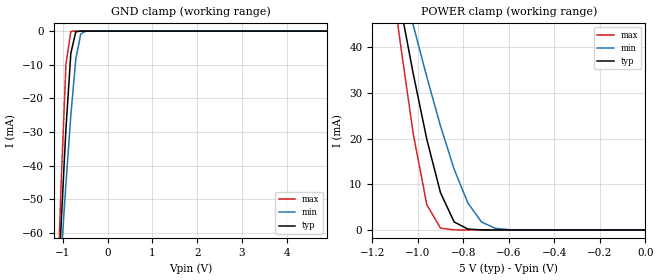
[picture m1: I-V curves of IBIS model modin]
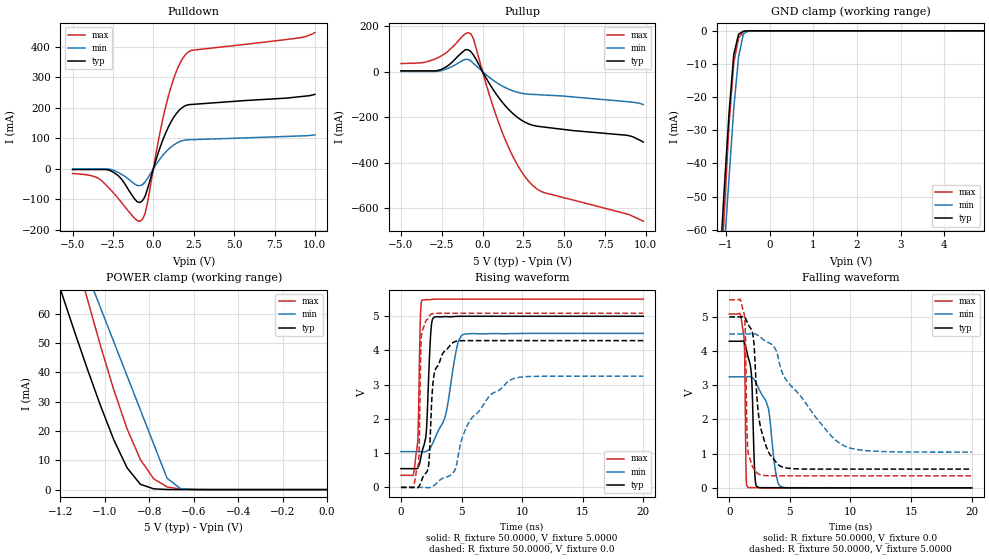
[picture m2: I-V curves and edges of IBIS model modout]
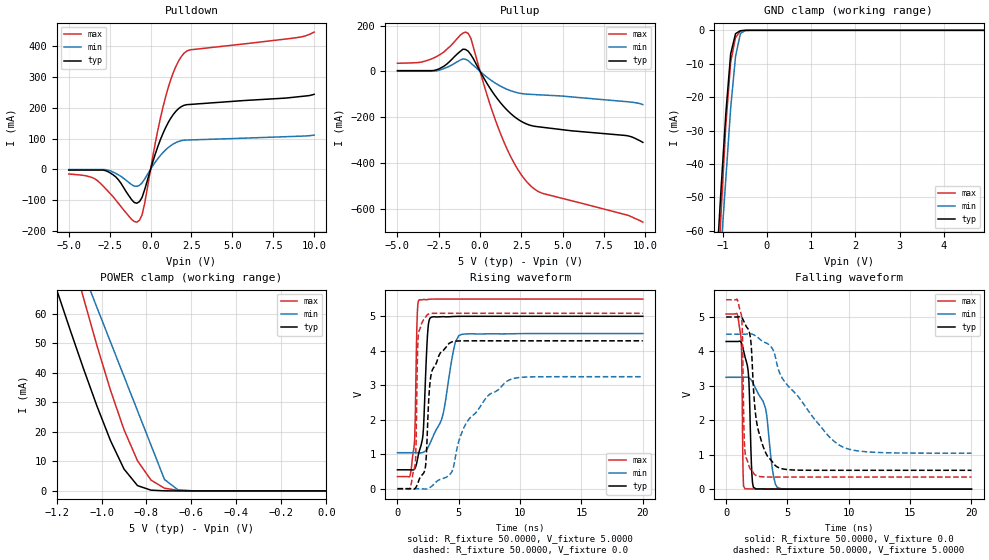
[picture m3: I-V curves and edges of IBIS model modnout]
| IBIS (I/O, Buffer, Information, Specification) Model, officially
| electronic behavioral standard for Buffer structures of digital pins.
[IBIS ver]  4.0
[File name] 54act74_5v0_rev1.ibs
[File Rev]  1.0
[Date]   18 July 2018
[Source]   CAD & Design Services (Catania) - STMicroelectronics
[Notes]
  (Note1) This IBIS model is the model of the product with package
   (Flat14 package elements);
  (Note2) This IBIS model is extracted with nominal 5.0V power supply
   (min:4.5V, typ:5.0V, max:5.5V);
  (Note3) This model has few Warnings about the non-monotonicity
   of I-V curves, but they are not indicative of problems
   inside the model;
|   Component 54ACT74
[Component] 54ACT74
[Manufacturer] STMicroelectronics
[Package]
| variable  typ   min   max
R_pkg   0.0   0.0   0.0
L_pkg   0.0H   0.0H   0.0H
C_pkg   0.0F   0.0F   0.0F
[Pin]   signal_name   model_name   R_pin   L_pin   C_pin
1   NCD1   modin   141.0m   4.31nH   1.01pF
2   D1   modin   108.1m   3.05nH   1.04pF
3   CP1   modin   90.5m   2.36nH   0.8pF
4   NSD1   modin   79.7m   1.96nH   0.8pF
5   Q1   modout   86.2m   2.16nH   0.8pF
6   NQ1   modnout   101.7m   2.85nH   1.04pF
7   GND   GND   111.0m   3.51nH   1.01pF
8   NQ2   modnout   141.0m   4.31nH   1.01pF
9   Q2   modout   112.4m   3.25nH   1.04pF
10   NSD2   modin   90.5m   2.36nH   0.8pF
11   CP2   modin   81.9m   2.06nH   0.8pF
12   D2   modin   84.0m   2.16nH   0.8pF
13   NCD2   modin   34.7m   0.86nH   0.80pF
14   VCC   POWER   111.0m   3.51nH   1.01pF
| Models and submodels in the file (3): modin (Input), modout (I/O), modnout (I/O)
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|   Model modin
[Model]   modin
Model_type Input
Vinl   =   1.500V
Vinh   =   3.500V
C_comp   0.532pF   0.404pF   0.702pF
[Temperature Range]  25.0000   0.1250k   -55.0000
[Voltage Range]   5.0000V   4.5000V   5.5000V
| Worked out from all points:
|   GND clamp passes 1 mA (typ) near -0.72 V on its own axis
|   POWER clamp passes 1 mA (typ) near -0.81 V on its own axis
[GND_clamp]
|Voltage   I(typ)   I(min)   I(max)
-5V       -1.28A     -953.7mA   -1.796A
-1.15V    -89.35mA   -90.45mA   -90.18mA
-1.04V    -58.19mA   -67.56mA   -46.36mA
-930mV    -29.16mA   -45.48mA   -9.95mA
-820mV    -6.597mA   -25mA      -92.8uA
-710mV    -202.6uA   -8.405mA   -269.9nA
-600mV    -2.872uA   -891.9uA   -789.3pA
-490mV    -39.72nA   -40.34uA   -15.19pA
4.9V      9.6pA      88.2pA     8.6pA
[POWER_clamp]
|Voltage   I(typ)   I(min)   I(max)
-4.98V    1.252A     928mA      1.764A
-1.14V    66.67mA    69.01mA    65.5mA
-1.08V    50.1mA     56.8mA     42.24mA
-1.02V    34.28mA    44.91mA    21.14mA
-960mV    19.83mA    33.48mA    5.531mA
-900mV    8.156mA    22.78mA    419.2uA
-840mV    1.752mA    13.29mA    18.09uA
-780mV    205.9uA    5.921mA    745.1nA
-720mV    20.4uA     1.757mA    30.64nA
-660mV    1.979uA    365.8uA    1.272nA
-600mV    191.5nA    66.17uA    65.13pA
0V        10pA       55.89pA    11pA
|   Model modout
[Model]   modout
Model_type I/O
Polarity   Inverting
Vinl   =   1.500V
Vinh   =   3.500V
Vmeas  =   2.500V
Cref   =   50pF
Rref   =   500
Vref   =   0
C_comp   2.793pF   2.323pF   3.682pF
[Temperature Range]   25.0000   0.1250k   -55.0000
[Voltage Range]   5.0000V   4.5000V   5.5000V
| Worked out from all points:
|   slope of the pulldown table from 0 to 0.75 V, typ, clamps not added: 6.47 ohm
|   slope of the pullup table from 0 to 0.75 V, typ, clamps not added: 8.35 ohm
|   GND clamp passes 1 mA (typ) near -0.71 V on its own axis
|   POWER clamp passes 1 mA (typ) near -0.81 V on its own axis
|   rising waveform, R_fixture 50.0000, V_fixture 5.0000: 20-80 % time 358ps typ, 1.26ns min, 174ps max; typ from 0.548 V to 5 V
|   rising waveform, R_fixture 50.0000, V_fixture 0.0: 20-80 % time 499ps typ, 2.57ns min, 156ps max; typ from 0 V to 4.29 V
|   falling waveform, R_fixture 50.0000, V_fixture 0.0: 20-80 % time 255ps typ, 818ps min, 106ps max; typ from 4.29 V to 0 V
|   falling waveform, R_fixture 50.0000, V_fixture 5.0000: 20-80 % time 784ps typ, 3.86ns min, 156ps max; typ from 5 V to 0.548 V
[Pulldown]
|Voltage   I(typ)   I(min)   I(max)
-5V       -2.551mA   -803.3uA   -15.35mA
-3.56V    -2.551mA   -803.3uA   -27.15mA
-2.6V     -7.851mA   -2.703mA   -71.53mA
-2.12V    -25.25mA   -13.48mA   -100.8mA
-1.16V    -98.75mA   -49.85mA   -162.8mA
-840mV    -110.5mA   -55.45mA   -172.2mA
-520mV    -91.67mA   -44.04mA   -148.4mA
440mV     73.46mA    34.38mA    126.4mA
920mV     135.7mA    63.13mA    236mA
1.4V      179.2mA    82.74mA    316.2mA
2.04V     208.1mA    94.66mA    377.2mA
10V       244mA      111.1mA    446.5mA
[Pullup]
|Voltage   I(typ)   I(min)   I(max)
-5V       3.588mA    923.3uA    35.83mA
-2.96V    3.588mA    923.3uA    54.38mA
-2.16V    24.35mA    13.48mA    87.04mA
-1.04V    97.31mA    54.56mA    167.5mA
-720mV    88.48mA    47.43mA    166.2mA
560mV     -69.07mA   -33.2mA    -135.3mA
1.36V     -147.6mA   -69.01mA   -294.6mA
2.16V     -202.5mA   -91.16mA   -413.9mA
2.96V     -233.7mA   -99.72mA   -493.1mA
3.76V     -243.9mA   -102.8mA   -532.4mA
8.88V     -280.6mA   -132.2mA   -627.5mA
9.84V     -310mA     -144.7mA   -658.8mA
[GND_clamp]
|Voltage   I(typ)   I(min)   I(max)
-5V       -1.024A    -833.9mA   -1.325A
-1.15V    -72.97mA   -87.27mA   -86.04mA
-1.04V    -48.13mA   -65.94mA   -55.47mA
-930mV    -25.02mA   -44.6mA    -28.46mA
-820mV    -7.036mA   -23.27mA   -9.536mA
-710mV    -1.004mA   -7.819mA   -2.181mA
-600mV    -110.4uA   -954.9uA   -202.2uA
-490mV    -9.508uA   -58.03uA   -7.172uA
-380mV    -722.1nA   -4.421uA   -237nA
4.9V      105.2pA    1.213nA    474pA
[POWER_clamp]
|Voltage   I(typ)   I(min)   I(max)
-4.98V    1.001A     830mA      1.314A
-1.2V     68.28mA    96.97mA    99.51mA
-1.14V    54.64mA    85.33mA    82.16mA
-1.08V    41.37mA    73.69mA    65.3mA
-1.02V    28.68mA    62.06mA    49.13mA
-960mV    17.02mA    50.42mA    34.07mA
-900mV    7.418mA    38.79mA    20.73mA
-840mV    1.802mA    27.15mA    10.21mA
-780mV    257.8uA    15.52mA    3.671mA
-720mV    36.76uA    3.879mA    913.2uA
-660mV    6.646uA    358.6uA    189.5uA
0V        111.1pA    0A         0A
[Ramp]
| variable   typ   min   max
dV/dt_r   2.5730/0.8335n   1.9489/2.6510n   3.0521/0.4316n
dV/dt_f   2.6714/0.8158n   2.0732/3.8408n   3.0891/0.3695n
R_load = 50.0000
[Rising Waveform]
R_fixture= 50.0000
V_fixture= 5.0000
V_fixture_min= 4.5000
V_fixture_max= 5.5000
|time   V(typ)   V(min)   V(max)
0s        547.7mV    1.045V     351.6mV
1.34ns    550.5mV    1.045V     1.186V
1.46ns    613.8mV    1.045V     2.203V
1.62ns    830.1mV    1.041V     5.097V
1.78ns    1.094V     1.038V     5.479V
2.08ns    1.561V     1.052V     5.484V
2.44ns    4.405V     1.165V     5.486V
2.68ns    4.957V     1.335V     5.496V
5ns       4.999V     4.442V     5.5V
20ns      5V         4.5V       5.5V
[Rising Waveform]
R_fixture= 50.0000
V_fixture= 0.0
V_fixture_min= 0.0
V_fixture_max= 0.0
|time   V(typ)   V(min)   V(max)
0s        145.2pV    0V         93.97pV
1.44ns    7.341mV    479.1uV    689.2mV
1.68ns    175.1mV    585.3uV    4.372V
2.28ns    632.7mV    -9.495mV   4.958V
2.48ns    2.054V     3.662mV    5.055V
2.8ns     3.397V     73.53mV    5.084V
4.44ns    4.258V     490.4mV    5.087V
5.64ns    4.288V     1.924V     5.087V
8.96ns    4.288V     3.125V     5.087V
20ns      4.288V     3.248V     5.087V
[Falling Waveform]
R_fixture= 50.0000
V_fixture= 0.0
V_fixture_min= 0.0
V_fixture_max= 0.0
|time   V(typ)   V(min)   V(max)
0s        4.288V     3.248V     5.087V
1.18ns    4.287V     3.248V     4.505V
1.26ns    4.234V     3.248V     4.017V
1.38ns    4.088V     3.248V     478.3mV
1.54ns    3.841V     3.252V     9.915mV
1.86ns    3.112V     3.233V     7.827mV
2.14ns    238.1mV    3.119V     7.774mV
2.42ns    8.301mV    2.913V     5.122mV
4.18ns    3.486mV    46.67mV    24.44uV
20ns      -2.477nV   887nV      -119.8nV
[Falling Waveform]
R_fixture= 50.0000
V_fixture= 5.0000
V_fixture_min= 4.5000
V_fixture_max= 5.5000
|time   V(typ)   V(min)   V(max)
0s        5V         4.5V       5.5V
1.24ns    5.004V     4.5V       5.064V
1.32ns    4.963V     4.499V     4.617V
1.44ns    4.876V     4.499V     1.934V
1.52ns    4.816V     4.5V       1.156V
2ns       4.344V     4.512V     572.3mV
2.36ns    2.311V     4.46V      414.9mV
4.12ns    656.1mV    3.668V     351.8mV
9.48ns    547.7mV    1.228V     351.6mV
20ns      547.7mV    1.045V     351.6mV
|   Model modnout
[Model]   modnout
Model_type I/O
Polarity   Non-Inverting
Vinl   =   1.500V
Vinh   =   3.500V
Vmeas  =   2.500V
Cref   =   50pF
Rref   =   500
Vref   =   0
C_comp   2.793pF   2.323pF   3.682pF
[Temperature Range]   25.0000   0.1250k   -55.0000
[Voltage Range]   5.0000V   4.5000V   5.5000V
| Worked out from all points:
|   slope of the pulldown table from 0 to 0.75 V, typ, clamps not added: 6.47 ohm
|   slope of the pullup table from 0 to 0.75 V, typ, clamps not added: 8.35 ohm
|   GND clamp passes 1 mA (typ) near -0.71 V on its own axis
|   POWER clamp passes 1 mA (typ) near -0.81 V on its own axis
|   rising waveform, R_fixture 50.0000, V_fixture 5.0000: 20-80 % time 358ps typ, 1.26ns min, 174ps max; typ from 0.548 V to 5 V
|   rising waveform, R_fixture 50.0000, V_fixture 0.0: 20-80 % time 499ps typ, 2.57ns min, 156ps max; typ from 0 V to 4.29 V
|   falling waveform, R_fixture 50.0000, V_fixture 0.0: 20-80 % time 255ps typ, 818ps min, 106ps max; typ from 4.29 V to 0 V
|   falling waveform, R_fixture 50.0000, V_fixture 5.0000: 20-80 % time 784ps typ, 3.86ns min, 156ps max; typ from 5 V to 0.548 V
[Pulldown]
|Voltage   I(typ)   I(min)   I(max)
-5V       -2.551mA   -803.3uA   -15.35mA
-3.56V    -2.551mA   -803.3uA   -27.15mA
-2.6V     -7.851mA   -2.703mA   -71.53mA
-2.12V    -25.25mA   -13.48mA   -100.8mA
-1.16V    -98.75mA   -49.85mA   -162.8mA
-840mV    -110.5mA   -55.45mA   -172.2mA
-520mV    -91.67mA   -44.04mA   -148.4mA
440mV     73.46mA    34.38mA    126.4mA
920mV     135.7mA    63.13mA    236mA
1.4V      179.2mA    82.74mA    316.2mA
2.04V     208.1mA    94.66mA    377.2mA
10V       244mA      111.1mA    446.5mA
[Pullup]
|Voltage   I(typ)   I(min)   I(max)
-5V       3.588mA    923.3uA    35.83mA
-2.96V    3.588mA    923.3uA    54.38mA
-2.16V    24.35mA    13.48mA    87.04mA
-1.04V    97.31mA    54.56mA    167.5mA
-720mV    88.48mA    47.43mA    166.2mA
560mV     -69.07mA   -33.2mA    -135.3mA
1.36V     -147.6mA   -69.01mA   -294.6mA
2.16V     -202.5mA   -91.16mA   -413.9mA
2.96V     -233.7mA   -99.72mA   -493.1mA
3.76V     -243.9mA   -102.8mA   -532.4mA
8.88V     -280.6mA   -132.2mA   -627.5mA
9.84V     -310mA     -144.7mA   -658.8mA
[GND_clamp]
|Voltage   I(typ)   I(min)   I(max)
-5V       -1.024A    -833.9mA   -1.325A
-1.15V    -72.97mA   -87.27mA   -86.04mA
-1.04V    -48.13mA   -65.94mA   -55.47mA
-930mV    -25.02mA   -44.6mA    -28.46mA
-820mV    -7.036mA   -23.27mA   -9.536mA
-710mV    -1.004mA   -7.819mA   -2.181mA
-600mV    -110.4uA   -954.9uA   -202.2uA
-490mV    -9.508uA   -58.03uA   -7.172uA
-380mV    -722.1nA   -4.421uA   -237nA
4.9V      105.2pA    1.213nA    474pA
[POWER_clamp]
|Voltage   I(typ)   I(min)   I(max)
-4.98V    1.001A     830mA      1.314A
-1.2V     68.28mA    96.97mA    99.51mA
-1.14V    54.64mA    85.33mA    82.16mA
-1.08V    41.37mA    73.69mA    65.3mA
-1.02V    28.68mA    62.06mA    49.13mA
-960mV    17.02mA    50.42mA    34.07mA
-900mV    7.418mA    38.79mA    20.73mA
-840mV    1.802mA    27.15mA    10.21mA
-780mV    257.8uA    15.52mA    3.671mA
-720mV    36.76uA    3.879mA    913.2uA
-660mV    6.646uA    358.6uA    189.5uA
0V        111.1pA    0A         0A
[Ramp]
| variable   typ   min   max
dV/dt_r   2.5730/0.8335n   1.9489/2.6510n   3.0521/0.4316n
dV/dt_f   2.6714/0.8158n   2.0732/3.8408n   3.0891/0.3695n
R_load = 50.0000
[Rising Waveform]
R_fixture= 50.0000
V_fixture= 5.0000
V_fixture_min= 4.5000
V_fixture_max= 5.5000
|time   V(typ)   V(min)   V(max)
0s        547.7mV    1.045V     351.6mV
1.34ns    550.5mV    1.045V     1.186V
1.46ns    613.8mV    1.045V     2.203V
1.62ns    830.1mV    1.041V     5.097V
1.78ns    1.094V     1.038V     5.479V
2.08ns    1.561V     1.052V     5.484V
2.44ns    4.405V     1.165V     5.486V
2.68ns    4.957V     1.335V     5.496V
5ns       4.999V     4.442V     5.5V
20ns      5V         4.5V       5.5V
[Rising Waveform]
R_fixture= 50.0000
V_fixture= 0.0
V_fixture_min= 0.0
V_fixture_max= 0.0
|time   V(typ)   V(min)   V(max)
0s        145.2pV    0V         93.97pV
1.44ns    7.341mV    479.1uV    689.2mV
1.68ns    175.1mV    585.3uV    4.372V
2.28ns    632.7mV    -9.495mV   4.958V
2.48ns    2.054V     3.662mV    5.055V
2.8ns     3.397V     73.53mV    5.084V
4.44ns    4.258V     490.4mV    5.087V
5.64ns    4.288V     1.924V     5.087V
8.96ns    4.288V     3.125V     5.087V
20ns      4.288V     3.248V     5.087V
[Falling Waveform]
R_fixture= 50.0000
V_fixture= 0.0
V_fixture_min= 0.0
V_fixture_max= 0.0
|time   V(typ)   V(min)   V(max)
0s        4.288V     3.248V     5.087V
1.18ns    4.287V     3.248V     4.505V
1.26ns    4.234V     3.248V     4.017V
1.38ns    4.088V     3.248V     478.3mV
1.54ns    3.841V     3.252V     9.915mV
1.86ns    3.112V     3.233V     7.827mV
2.14ns    238.1mV    3.119V     7.774mV
2.42ns    8.301mV    2.913V     5.122mV
4.18ns    3.486mV    46.67mV    24.44uV
20ns      -2.477nV   887nV      -119.8nV
[Falling Waveform]
R_fixture= 50.0000
V_fixture= 5.0000
V_fixture_min= 4.5000
V_fixture_max= 5.5000
|time   V(typ)   V(min)   V(max)
0s        5V         4.5V       5.5V
1.24ns    5.004V     4.5V       5.064V
1.32ns    4.963V     4.499V     4.617V
1.44ns    4.876V     4.499V     1.934V
1.52ns    4.816V     4.5V       1.156V
2ns       4.344V     4.512V     572.3mV
2.36ns    2.311V     4.46V      414.9mV
4.12ns    656.1mV    3.668V     351.8mV
9.48ns    547.7mV    1.228V     351.6mV
20ns      547.7mV    1.045V     351.6mV
